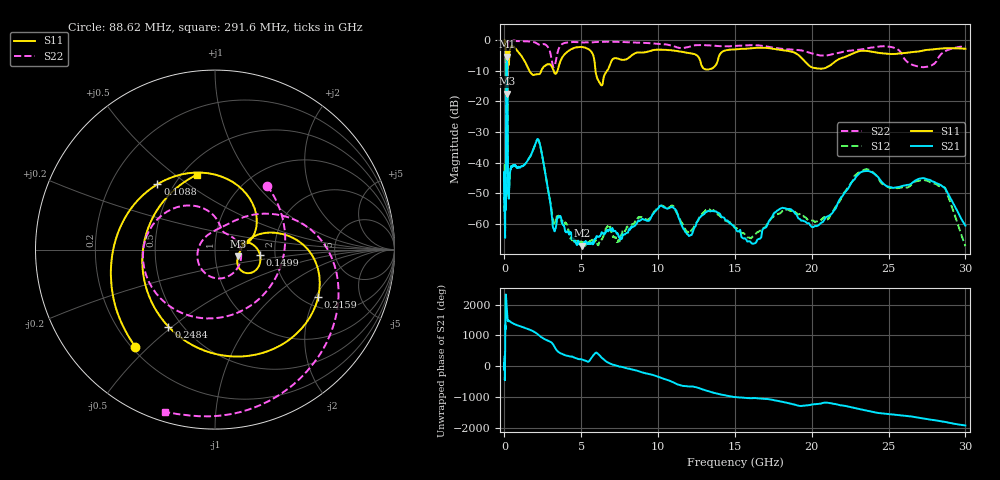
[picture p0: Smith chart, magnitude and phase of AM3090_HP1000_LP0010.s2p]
! Date/Time: Thu, Feb 28, 2019 2:01 PM
! Network Analyzer: Agilent Technologies E8364B Rev: A.07.50.67
! Sweep from 0.010 to 30.000 GHz, 1601 Points, Sweep Type: LOG
! Power Supply: 5.022 V, 0.002 A
# Hz S DB R 50
!freq MagS11 AngS11 MagS21 AngS21 MagS12 AngS12 MagS22 AngS22
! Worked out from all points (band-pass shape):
!   1601 points, 10 MHz to 30 GHz, reference 50 ohm
!   highest |S21| = -5.43 dB at 149.1 MHz (marker M1); lowest = -67.0 dB at 5.027 GHz (marker M2)
!   |S21| within 3 dB of the highest: 121.3 MHz to 186.8 MHz (65.41 MHz wide, 42.5 % of centre)
!   lowest |S11| = -17.5 dB at 184 MHz (marker M3), VSWR 1.31, Z = 64.6 - j4.84 ohm
!   |S11| at or under -10 dB: 1.619 GHz to 2.398 GHz (779.6 MHz wide, 38.8 % of centre); 3.201 GHz to 3.454 GHz (253.6 MHz wide, 7.62 % of centre); 5.925 GHz to 6.693 GHz (767.4 MHz wide, 12.2 % of centre)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
!   |S22| runs from -21.3 to -0.2 dB; largest |S21 - S12| = 0.016
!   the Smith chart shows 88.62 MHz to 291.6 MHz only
!   S11 on the Smith chart (normalised r, x): 88.62 MHz: 0.21, -0.45; 108.8 MHz: 0.41, +0.39; 149.9 MHz: 1.66, -0.10; 215.9 MHz: 2.38, -2.11; 248.4 MHz: 0.42, -0.48; 291.6 MHz: 0.59, +0.60
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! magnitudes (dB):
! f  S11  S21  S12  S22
! 10 MHz  -0.2  -43.2  -40.6  -0.6
! 38.04 MHz  -0.5  -58.9  -58.9  -1.3
! 88.62 MHz  -3.1  -50.7  -49.8  -6.8
! 108.8 MHz  -6.3  -19.8  -19.8  -7.8
! 144.7 MHz  -12.8  -5.4  -5.4  -17.2
! 149.1 MHz  -12.1  -5.4  -5.4  -16.3
! 149.9 MHz  -12.0  -5.4  -5.4  -16.2
! 184 MHz  -17.5  -7.7  -7.7  -20.2
! 215.9 MHz  -4.0  -43.3  -42.8  -2.8
! 248.4 MHz  -6.0  -49.6  -48.9  -0.9
! 291.6 MHz  -7.4  -50.6  -49.1  -0.5
! 550.5 MHz  -2.1  -41.0  -41.1  -0.3
! 2.084 GHz  -11.2  -32.9  -32.9  -1.0
! 3.22 GHz  -10.3  -61.8  -59.8  -8.8
! 5.027 GHz  -2.3  -67.0  -66.5  -0.8
! 6.202 GHz  -14.0  -63.9  -65.4  -0.6
! 7.926 GHz  -6.3  -63.0  -61.6  -0.7
! 10.49 GHz  -3.2  -54.8  -54.6  -1.4
! 16.05 GHz  -2.7  -66.1  -64.6  -1.7
! 23.48 GHz  -3.5  -42.7  -42.1  -2.9
! 27.83 GHz  -3.1  -46.0  -46.6  -8.2
! 30 GHz  -2.9  -60.5  -67.2  -2.2
